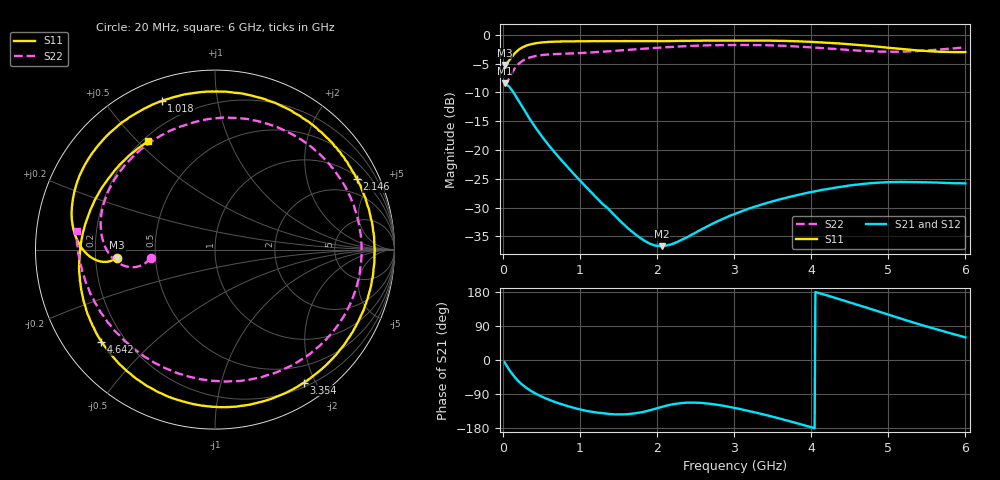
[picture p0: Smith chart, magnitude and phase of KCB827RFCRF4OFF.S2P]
!Agilent Technologies,E5071B,JP1KK00126,A.08.11
!Date: Tue May 06 07:16:46 2014
!Data & Calibration Information:
!Freq	S11:SOLT2(ON)	S21:SOLT2(ON)	S12:SOLT2(ON)	S22:SOLT2(ON)
# Hz S dB R 50
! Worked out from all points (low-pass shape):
!   600 points, 20 MHz to 6 GHz, reference 50 ohm
!   highest |S21| = -8.43 dB at 20 MHz (marker M1); lowest = -36.7 dB at 2.057 GHz (marker M2)
!   |S21| within 3 dB of the highest: start of sweep to 201.2 MHz
!   lowest |S11| = -5.2 dB at 20 MHz (marker M3), VSWR 3.41, Z = 14.7 - j1.86 ohm
!   |S11| at or under -10 dB: nowhere
!   |S22| runs from -8.9 to -1.7 dB; largest |S21 - S12| = 0.00093
!   S11 on the Smith chart (normalised r, x): 20 MHz: 0.29, -0.04; 1.018 GHz: 0.10, +0.70; 2.146 GHz: 1.10, +3.96; 3.354 GHz: 0.26, -1.85; 4.642 GHz: 0.11, -0.35; 6 GHz: 0.22, +0.54
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2e7  -5.24 -175.4  -8.43 -5.9  -8.42 -5.9  -8.87 -172.8
1.597663e8  -3.10 -176.9  -10.53 -47.1  -10.51 -47.1  -5.67 -170.3
2.795659e8  -1.99 172.1  -13.19 -70.1  -13.18 -70.1  -4.30 179.1
4.093489e8  -1.50 159.8  -15.88 -87.2  -15.86 -87.2  -3.71 167.6
7.088481e8  -1.17 134.1  -21.03 -113.5  -21.02 -113.5  -3.31 144.9
1.018331e9  -1.12 109.7  -25.58 -131.2  -25.57 -131.3  -3.16 123.4
1.25793e9  -1.10 91.6  -28.92 -139.7  -28.92 -139.6  -2.97 107.0
1.497529e9  -1.09 73.7  -32.03 -143.9  -32.02 -143.7  -2.73 90.9
1.747112e9  -1.09 55.3  -34.93 -139.8  -34.94 -139.5  -2.49 73.8
2.016661e9  -1.08 35.8  -36.63 -126.2  -36.66 -126.0  -2.23 56.0
2.056594e9  -1.08 33.0  -36.70 -123.9  -36.70 -123.9  -2.20 53.4
2.146444e9  -1.08 26.5  -36.51 -119.2  -36.51 -119.3  -2.12 47.8
2.58571e9  -1.00 -4.3  -33.70 -113.4  -33.71 -113.7  -1.85 22.0
3.014992e9  -0.99 -33.8  -31.04 -127.0  -31.05 -127.0  -1.76 -0.6
3.354424e9  -1.00 -56.2  -29.48 -142.5  -29.48 -142.5  -1.79 -17.5
3.683873e9  -1.06 -77.5  -28.26 -159.7  -28.23 -159.8  -1.92 -34.3
4.013322e9  -1.23 -98.8  -27.26 -178.2  -27.25 -178.1  -2.18 -52.5
4.312821e9  -1.46 -118.6  -26.53 163.8  -26.52 163.7  -2.45 -71.3
4.64227e9  -1.78 -140.9  -25.93 142.9  -25.93 143.1  -2.76 -94.4
5.011653e9  -2.25 -167.1  -25.58 118.9  -25.58 119.0  -2.93 -122.5
5.510818e9  -2.83 156.5  -25.62 87.7  -25.61 87.8  -2.71 -158.8
6e9  -2.98 121.6  -25.80 59.6  -25.82 59.9  -2.18 172.5
